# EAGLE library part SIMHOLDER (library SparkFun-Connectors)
SIM Socket Socket for SIM cellular cards. Schematic element and footprint production proven. Spark Fun Electronics SKU : PRT-00548
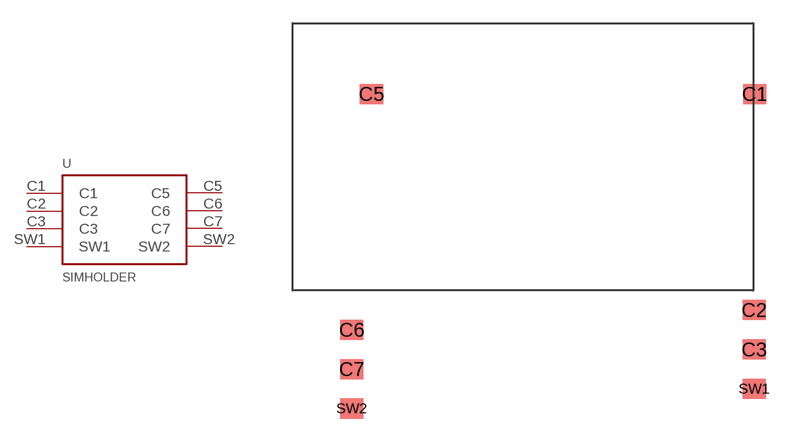
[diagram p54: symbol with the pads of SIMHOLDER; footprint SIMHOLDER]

Designator prefix -

## SIMHOLDER  [SIMHOLDER]
C1  C1
C2  C2
C3  C3
C5  C5
C6  C6
C7  C7
SW1  SW1
SW2  SW2

## Footprint SIMHOLDER (pad centres in mm)
smd 1.5 x 1.3: C1 29.81,12.7; C2 29.78,-1.26; C3 29.78,-3.81; C5 5.08,12.7; C6 3.81,-2.54; C7 3.81,-5.08; SW1 29.78,-6.35; SW2 3.81,-7.62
